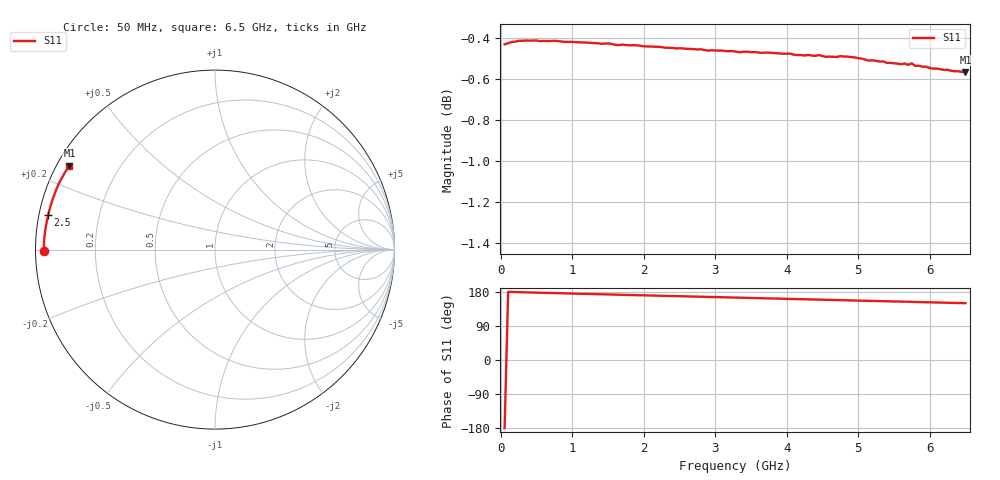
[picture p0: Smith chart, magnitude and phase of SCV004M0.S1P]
! Infineon Technologies  Discrete & RF Semiconductors
! BAR63-02L
! Si PIN Diode in TSLP-2
! IF = 4 mA
! S-Parameters:  March  2002
# GHz  S  MA  R  50
!  f  S11
! GHz  MAG  ANG
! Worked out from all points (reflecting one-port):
!   130 points, 50 MHz to 6.5 GHz, reference 50 ohm
!   lowest |S11| = -0.6 dB at 6.5 GHz (marker M1), VSWR 30.66, Z = 1.75 + j13.4 ohm
!   phase of S11 starts at -179 deg and turns -31 deg over the sweep
!   S11 on the Smith chart (normalised r, x): 50 MHz: 0.02, -0.01; 2.5 GHz: 0.03, +0.10; 6.5 GHz: 0.03, +0.27
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0.05  0.9515 -179.4
0.1  0.9521 180.0
0.15  0.9527 179.6
0.25  0.9534 179.0
0.6  0.9533 177.2
0.7  0.9533 176.8
0.9  0.9528 175.8
1.25  0.9522 174.1
1.65  0.9511 172.3
1.7  0.9513 172.0
2.5  0.9494 168.3
2.9  0.9481 166.5
2.95  0.9483 166.2
3.1  0.9481 165.6
3.3  0.9475 164.6
3.45  0.9475 164.0
4.1  0.9459 160.9
4.25  0.9455 160.3
4.45  0.9458 159.3
4.6  0.945 158.7
4.9  0.9447 157.2
5.3  0.9424 155.4
5.35  0.9424 155.1
5.7  0.9406 153.6
5.75  0.9414 153.4
5.8  0.94 153.1
5.95  0.9397 152.4
6.5  0.9368 150.0
